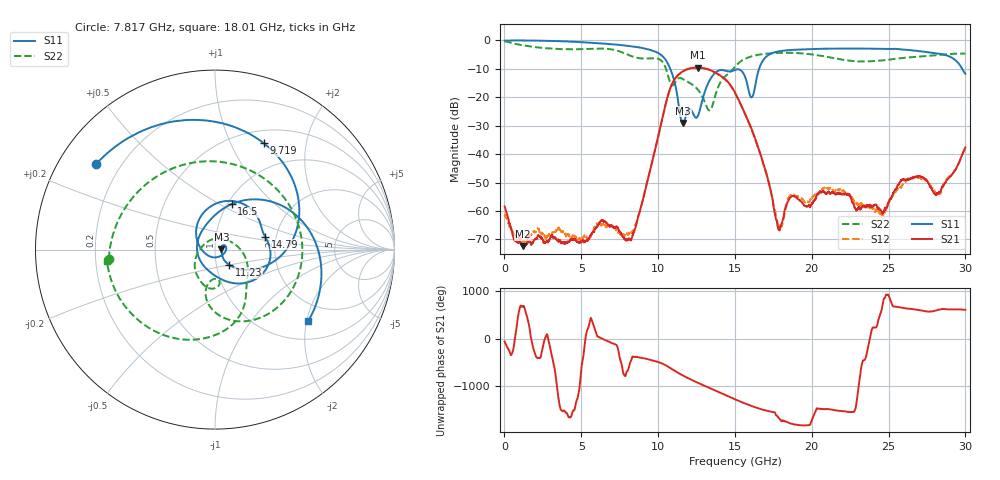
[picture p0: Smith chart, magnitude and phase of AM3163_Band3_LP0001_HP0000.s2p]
!Agilent Technologies,E8364B,MY43040894,A.07.50.67
!Agilent E8364B: A.07.50.67
!Date: Thursday, August 20, 2020 12:13:13
!Correction: S11(Full 2 Port(1,2))
!S21(Full 2 Port(1,2))
!S12(Full 2 Port(1,2))
!S22(Full 2 Port(1,2))
!S2P File: Measurements: S11, S21, S12, S22:
# Hz S  dB  R 50
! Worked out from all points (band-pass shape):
!   3201 points, 10 MHz to 30 GHz, reference 50 ohm
!   highest |S21| = -9.55 dB at 12.57 GHz (marker M1); lowest = -72.4 dB at 1.191 GHz (marker M2)
!   |S21| within 3 dB of the highest: 11.23 GHz to 14.11 GHz (2.878 GHz wide, 22.7 % of centre)
!   lowest |S11| = -29.0 dB at 11.63 GHz (marker M3), VSWR 1.07, Z = 53.6 + j0.3 ohm
!   |S11| at or under -10 dB: 10.79 GHz to 16.57 GHz (5.776 GHz wide, 42.2 % of centre); 29.79 GHz to end of sweep
!   |S22| runs from -24.6 to -0.3 dB; largest |S21 - S12| = 0.0047
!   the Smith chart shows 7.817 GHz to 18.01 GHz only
!   S11 on the Smith chart (normalised r, x): 7.817 GHz: 0.11, +0.32; 9.719 GHz: 0.65, +1.35; 11.23 GHz: 1.15, -0.20; 14.79 GHz: 1.74, +0.28; 16.5 GHz: 1.05, +0.57; 18.01 GHz: 1.47, -2.05
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1e7  -0.02 -1.9  -58.40 -63.3  -61.71 -25.6  -0.31 -7.2
1.190856e9  -0.01 -32.7  -72.38 -36.8  -70.79 58.0  -1.72 -102.8
2.643497e9  -0.11 -72.4  -70.90 3.9  -69.11 -91.7  -2.70 167.7
5.014581e9  -0.61 -135.6  -70.62 117.5  -69.67 134.8  -3.07 41.8
6.75775e9  -1.23 176.5  -64.85 -60.0  -64.90 -65.9  -2.99 -76.7
7.816772e9  -1.77 144.1  -69.81 -54.0  -68.56 53.4  -4.53 -175.1
8.688356e9  -2.38 113.0  -62.09 -32.9  -62.50 -35.8  -6.16 91.2
9.719262e9  -3.72 65.3  -40.31 -106.9  -40.39 -107.8  -6.25 -14.0
1.000979e10  -4.43 47.6  -33.64 -136.0  -33.81 -136.8  -6.49 -43.0
1.122813e10  -18.66 -47.2  -12.59 8.6  -12.66 8.6  -13.78 -84.9
1.163112e10  -29.05 4.5  -10.78 -64.0  -10.88 -63.9  -13.63 -107.0
1.256831e10  -26.77 -117.9  -9.55 147.8  -9.59 148.1  -17.19 -144.7
1.352424e10  -12.57 98.7  -10.74 11.2  -10.79 10.7  -23.15 61.1
1.478945e10  -10.81 14.6  -16.33 -171.6  -16.53 -171.6  -10.54 -54.2
1.5005e10  -10.36 4.0  -18.33 156.3  -18.54 156.5  -9.26 -61.3
1.649513e10  -11.37 69.9  -37.19 -31.8  -37.50 -30.0  -5.07 -122.5
1.801337e10  -3.68 -37.4  -64.76 59.0  -65.66 -132.1  -4.35 -173.8
2.000958e10  -3.01 -100.2  -57.22 80.5  -55.41 -23.4  -4.92 116.5
2.242752e10  -2.82 -156.2  -54.25 -112.3  -54.41 -121.0  -7.12 9.2
2.500479e10  -3.00 144.2  -57.00 -169.1  -57.02 -30.6  -6.80 -105.5
2.73665e10  -3.99 78.7  -48.71 -141.7  -48.91 -138.5  -5.51 174.5
3e10  -11.73 -28.8  -37.63 -114.3  -38.04 -115.2  -4.61 98.2
